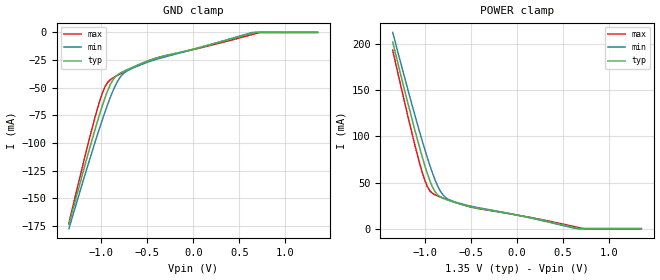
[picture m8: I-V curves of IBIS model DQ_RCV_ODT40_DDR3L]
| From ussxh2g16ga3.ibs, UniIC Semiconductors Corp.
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|   Model DQ_RCV_ODT40_DDR3L
[Model] DQ_RCV_ODT40_DDR3L
Model_type Input
Vinl =  0.540V
Vinh =  0.810V
C_comp   0.966pF   0.965pF   0.967pF
[Model Spec]
Vinh   0.810V   0.776V   0.860V
Vinl   0.540V   0.506V   0.590V
[Temperature Range]   25.000   95.000   -40.000
[Voltage Range]   1.350V   1.283V   1.450V
[GND_clamp]
|Voltage   I(typ)   I(min)   I(max)
-1.35V    -173.6mA   -177.4mA   -172.2mA
-1.154V   -113.3mA   -122.7mA   -104.7mA
-1.014V   -73.19mA   -85.62mA   -61.52mA
-958mV    -58.96mA   -71.76mA   -48.99mA
-930mV    -52.69mA   -65.19mA   -45.13mA
-874mV    -43.07mA   -53.18mA   -41.2mA
-818mV    -38.08mA   -43.58mA   -38.65mA
-734mV    -34.31mA   -35.63mA   -35.08mA
-482mV    -25.44mA   -26.56mA   -25.57mA
638mV     -757.9uA   -84.43uA   -1.992mA
750mV     0A         0A         0A
1.35V     0A         0A         0A
[POWER_clamp]
|Voltage   I(typ)   I(min)   I(max)
-1.35V    202.4mA    212.8mA    193.5mA
-1.114V   108.6mA    124.8mA    92.51mA
-1.058V   87.93mA    105mA      71mA
-1.002V   68.6mA     86.08mA    52.58mA
-946mV    51.85mA    68.39mA    40.95mA
-890mV    40.02mA    52.83mA    36.68mA
-834mV    34.46mA    40.91mA    34.39mA
-778mV    31.93mA    33.98mA    32.3mA
-526mV    24.31mA    24.99mA    24.09mA
650mV     678.6uA    0A         1.63mA
734mV     0A         0A         0A
1.35V     0A         0A         0A
